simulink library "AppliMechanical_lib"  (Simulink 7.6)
settings: Solver=ode45  StartTime=0.0  StopTime=10.0  RelTol=1e-3
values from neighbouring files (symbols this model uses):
  A = [1+j -(1-j);1 -2/(1-j)]    [systeme_AX_B_phaseurs.m]
  m = 10    [masse_ressort_enveloppe.m]
  N = 50;')    [Prog_callbacks.m]    (also in _startup.m = 0.001'))
undefined symbols (not defined in the file or in its folder): AppliMechanical, Charge_mecanique, DC_Moteur_serie, gcbh, H, kg, nesl_callback, Ohm, rad, s

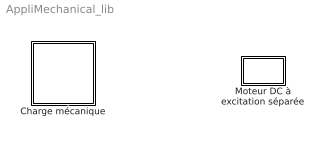
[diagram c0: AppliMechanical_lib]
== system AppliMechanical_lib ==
  Charge mécanique : Subsystem  DialogController=NetworkEngine.DynNeDlgSource  LoadFcn=nesl_callback('LoadFcn',gcbh);  mask(Charge mécanique){ComponentPath=AppliMechanical.Charge_mecanique, ClassName=Charge_mecanique, SchemaVersion=1, k=10, k_unit=N*m/rad, J=0.01, J_unit=kg*m^2, fr=0.01, fr_unit=N*m/(rad/s), alpha_Log=off, t_Log=off, w_Log=off, LocalVarNames=\, LocalVarDescs=alpha\, LocalVarLogging=t\}
      mask prompts: k "raideur du ressort"; J "couple d'inertie"; fr "frottements visqueux"
      mask help: Inertie J, frottements fr, ressort de raideur k
      mask init:
      | nesl_preinitmask (gcb);
  Moteur DC à excitation séparée : Subsystem  DialogController=NetworkEngine.DynNeDlgSource  LoadFcn=nesl_callback('LoadFcn',gcbh);  mask(Moteur DC à
excitation séparée){ComponentPath=AppliMechanical.DC_Moteur_serie, ClassName=DC_Moteur_serie, SchemaVersion=1, K=0.1, K_unit=N*m/A, Ri=4.9, Ri_unit=Ohm, Li=1e-5, Li_unit=H, fr=0.02, fr_unit=N*m/(rad/s), J=1e-5, J_unit=kg*m^2, w_Log=off, i_Log=off, v_Log=off, t_Log=off, LocalVarNames=\, LocalVarDescs=w\, LocalVarLogging=i\}
      mask prompts: K "Constante de proportionalité K"; Ri "Résistance d'induit"; Li "inductance d'induit"; fr "couple de frottement"; J "moment d'inertie"
      mask init:
      | nesl_preinitmask (gcb);

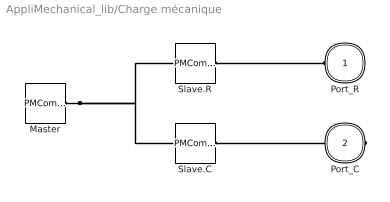
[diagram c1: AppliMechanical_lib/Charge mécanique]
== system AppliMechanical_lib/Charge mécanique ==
  Master : PMComponent  Tag=AppliMechanical.Charge_mecanique  PhysicalDomain=network_engine_domain  SubClassName=master  LeftPortType=generic  RightPortType=generic  RConnTagsString=RConn1
  Slave.C : PMComponent  Tag=C  PhysicalDomain=network_engine_domain  SubClassName=terminal  LeftPortType=generic  RightPortType=foundation.mechanical.rotational.rotational  LConnTagsString=LConn1  RConnTagsString=RConn1
  Slave.R : PMComponent  Tag=R  PhysicalDomain=network_engine_domain  SubClassName=terminal  LeftPortType=generic  RightPortType=foundation.mechanical.rotational.rotational  LConnTagsString=LConn1  RConnTagsString=RConn1
  Port_R : PMIOPort  Tag=R  Port=1  Side=Left
  Port_C : PMIOPort  Tag=C  Port=2  Side=Right
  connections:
  Slave.R/RConn1 -- Port_R/RConn1
  Master/RConn1 -- Slave.R/LConn1 -- Slave.C/LConn1
  Slave.C/RConn1 -- Port_C/RConn1

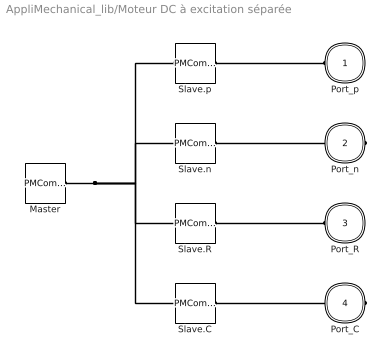
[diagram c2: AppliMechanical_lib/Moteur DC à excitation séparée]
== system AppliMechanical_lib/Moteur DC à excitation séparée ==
  Master : PMComponent  Tag=AppliMechanical.DC_Moteur_serie  PhysicalDomain=network_engine_domain  SubClassName=master  LeftPortType=generic  RightPortType=generic  RConnTagsString=RConn1
  Slave.C : PMComponent  Tag=C  PhysicalDomain=network_engine_domain  SubClassName=terminal  LeftPortType=generic  RightPortType=foundation.mechanical.rotational.rotational  LConnTagsString=LConn1  RConnTagsString=RConn1
  Slave.R : PMComponent  Tag=R  PhysicalDomain=network_engine_domain  SubClassName=terminal  LeftPortType=generic  RightPortType=foundation.mechanical.rotational.rotational  LConnTagsString=LConn1  RConnTagsString=RConn1
  Slave.n : PMComponent  Tag=n  PhysicalDomain=network_engine_domain  SubClassName=terminal  LeftPortType=generic  RightPortType=foundation.electrical.electrical  LConnTagsString=LConn1  RConnTagsString=RConn1
  Slave.p : PMComponent  Tag=p  PhysicalDomain=network_engine_domain  SubClassName=terminal  LeftPortType=generic  RightPortType=foundation.electrical.electrical  LConnTagsString=LConn1  RConnTagsString=RConn1
  Port_p : PMIOPort  Tag=p  Port=1  Side=Left
  Port_n : PMIOPort  Tag=n  Port=2  Side=Right
  Port_R : PMIOPort  Tag=R  Port=3  Side=Left
  Port_C : PMIOPort  Tag=C  Port=4  Side=Right
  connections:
  Slave.p/RConn1 -- Port_p/RConn1
  Slave.p/LConn1 -- Slave.n/LConn1 -- Slave.R/LConn1 -- Master/RConn1 -- Slave.C/LConn1
  Slave.n/RConn1 -- Port_n/RConn1
  Slave.R/RConn1 -- Port_R/RConn1
  Slave.C/RConn1 -- Port_C/RConn1
